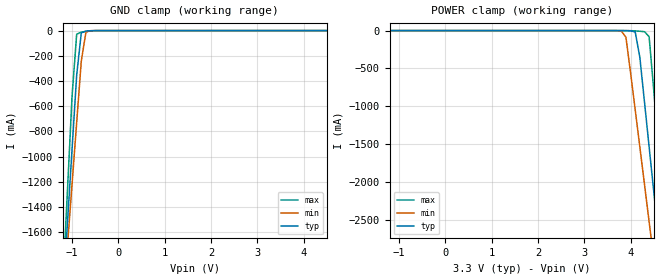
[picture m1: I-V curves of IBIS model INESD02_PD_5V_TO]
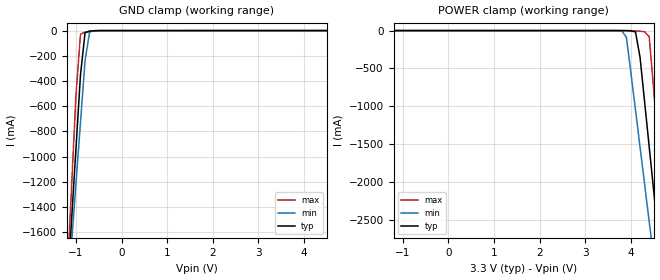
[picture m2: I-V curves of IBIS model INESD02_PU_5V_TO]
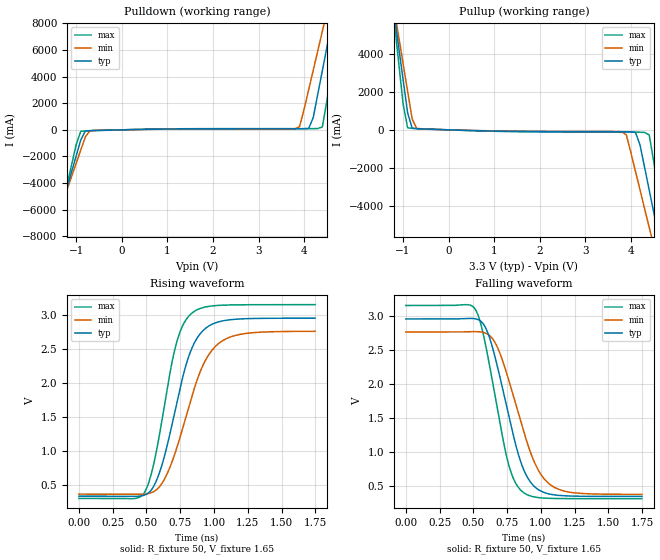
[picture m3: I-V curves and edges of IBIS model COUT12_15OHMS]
|   This file is an IBIS representation of the   |
|   Integrated Device Technology, Inc.   |
|   ICS810252i-02   |
[IBIS Ver]   4.1
[File name]   810252di_02_3v3.ibs
[File Rev]   1.0
[Date]   28 Apr 2009 | Last modified
|   Nov 27 2007  | Generated
[Source]   Originated at Integrated Devices Technology, Inc.
[Disclaimer]
IDT hereby grants the user of this IBIS model a non-exclusive,
nontransferable license to use this IBIS model under the following terms.
Before using this IBIS model, the user should read this license.
If the user does not accept these terms,  the IBIS model should be
returned to IDT within 30 days.
   The user is granted this license only to use the IBIS model and
is not granted rights to sell, load, rent, lease or license the IBIS
model in whole or in part, or in modified form to anyone other than
user. User may modify the IBIS model to suit its specific
applications but rights to derivative works and such modifications
shall belong to IDT.
   This IBIS model is provided on an "AS IS" basis and IDT makes
absolutely no warranty with respect to the information contained
herein. IDT DISCLAIMS AND CUSTOMER WAIVES ALL WARRANTIES, EXPRESS
OR IMPLIED, INCLUDING WARRANTIES OF MERCHANTABILITY OR FITNESS FOR
A PARTICULAR PURPOSE. The entire risk as to quality and performance
is with the Customer. ACCORDINGLY, IN NO EVENT SHALL THE COMPANY BE
LIABLE FOR ANY DAMAGES, WHETHER IN CONTRACT OR TORT,INCLUDING ANY
LOST PROFITS OR OTHER INCIDENTAL, CONSEQUENTIAL, EXEMPLARY, OR
PUNITIVE DAMAGES ARISING OUT OF THE USE OR APPLICATION OF THE IBIS
model provided in this package. Further, IDT reserves the right to
make changes without notice to any product herein to improve
reliability, function, or design. IDT does not convey any license
under patent rights or any other intellectual property rights,
including those of third parties.
   IDT is not obligated to provide maintenance or support
for the licensed IBIS model.
[Copyright]   Copyright 2007 by Integrated Device Technology, Inc.
[Component]   ICS810252DKI-02
[Manufacturer] Integrated Devices Technology, Inc.
[Package]
|QFN 32
|lead + wire   typ   min   max
R_pkg   72.4655m   58.886m   86.045m
L_pkg   1.47175nH   1.11650nH   1.77850nH
C_pkg   0.07747pF   0.07444pF   0.08050pF
[Pin] signal_name   model_name   R_pin   L_pin   C_pin
1   LF1   NC   86.045m   1.77850nH   0.08050pF
2   LF0   NC   76.996m   1.55783nH   0.07848pF
3   ISET   NC   67.941m   1.33717nH   0.07646pF
4   GND   GND   58.886m   1.11650nH   0.07444pF
5   CLK_SEL   INESD02_PD_5V_TO   58.886m   1.11650nH   0.07444pF
6   VDD   POWER   67.941m   1.33717nH   0.07646pF
7   RESERVED   NC   76.996m   1.55783nH   0.07848pF
8   GND   GND   86.045m   1.77850nH   0.08050pF
9   PDSEL_2   INESD02_PU_5V_TO   86.045m   1.77850nH   0.08050pF
10   PDSEL_1   INESD02_PU_5V_TO   76.996m   1.55783nH   0.07848pF
11   PDSEL_0   INESD02_PU_5V_TO   67.941m   1.33717nH   0.07646pF
12   VDD   POWER   58.886m   1.11650nH   0.07444pF
13   VDDA   POWER   58.886m   1.11650nH   0.07444pF
14   ODBSEL_1   INESD02_PD_5V_TO   67.941m   1.33717nH   0.07646pF
15   ODBSEL_0   INESD02_PD_5V_TO   76.996m   1.55783nH   0.07848pF
16   ODASEL_1   INESD02_PD_5V_TO   86.045m   1.77850nH   0.08050pF
17   ODASEL_0   INESD02_PD_5V_TO   86.045m   1.77850nH   0.08050pF
18   GND   GND   76.996m   1.55783nH   0.07848pF
19   QA   COUT12_15OHMS   67.941m   1.33717nH   0.07646pF
20   NC   NC   58.886m   1.11650nH   0.07444pF
21   VDDO   POWER   58.886m   1.11650nH   0.07444pF
22   QB   COUT12_15OHMS   67.941m   1.33717nH   0.07646pF
23   NC   NC   76.996m   1.55783nH   0.07848pF
24   GND   GND   86.045m   1.77850nH   0.08050pF
25   nCLK1   INESD02_PMID_5V_   86.045m   1.77850nH   0.08050pF
26   CLK1   INESD02_PD_5V_TO   76.996m   1.55783nH   0.07848pF
27   VDD   POWER   67.941m   1.33717nH   0.07646pF
28   nCLK0   INESD02_PMID_5V_   58.886m   1.11650nH   0.07444pF
29   CLK0   INESD02_PD_5V_TO   58.886m   1.11650nH   0.07444pF
30   XTAL_OUT   NC   67.941m   1.33717nH   0.07646pF
31   XTAL_IN   NC   76.996m   1.55783nH   0.07848pF
32   VDDX   POWER   86.045m   1.77850nH   0.08050pF
| Models and submodels in the file (4): INESD02_PD_5V_TO (Input), INESD02_PU_5V_TO (Input), COUT12_15OHMS (Output), INESD02_PMID_5V_ (Input)
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[Model]   INESD02_PD_5V_TO
Model_type   Input
Polarity   Non-Inverting
Vinl = 0.8V
Vinh = 2.0V
|   typ   min   max
C_comp   2pF   1.5pF   2.5pF
|   typ   min   max
[Voltage range]  3.3V   3.135V   3.465V
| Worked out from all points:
|   GND clamp passes 1 mA (typ) near -0.60 V on its own axis
[GND_clamp]
|Voltage I(typ)   I(min)   I(max)
-3.3V     -14.52A    -12.53A    -17.87A
-1.2V     -2.123A    -2.201A    -2.031A
-1.1V     -1.533A    -1.71A     -1.276A
-1V       -943mA     -1.22A     -522mA
-900mV    -353.5mA   -729.8mA   -28.69mA
-800mV    -17.79mA   -240.3mA   -12.18mA
-700mV    -3.491mA   -12mA      -6.618mA
-600mV    -1.033mA   -835uA     -2.43mA
6.6V      128.6uA    160.8uA    121.8uA
[POWER_clamp]
|Voltage   I(typ)   I(min)   I(max)
-3.3V     128.6uA    156.8uA    124.8uA
3.8V      -180.1uA   -4.403mA   -11.05uA
3.9V      -1.033mA   -88.76mA   -99.86uA
4.1V      -17.79mA   -1.048A    -3.685mA
4.2V      -353.5mA   -1.539A    -8.437mA
4.3V      -943mA     -2.029A    -14.61mA
4.4V      -1.533A    -2.52A     -80.08mA
4.5V      -2.123A    -3.011A    -786mA
4.6V      -2.713A    -3.502A    -1.54A
4.7V      -3.303A    -3.994A    -2.295A
4.8V      -3.894A    -4.485A    -3.049A
6.6V      -14.52A    -13.34A    -16.62A
[Model]   INESD02_PU_5V_TO
Model_type   Input
Polarity   Non-Inverting
Vinl = 1.4V
Vinh = 1.85V
|   typ   min   max
C_comp   2pF   1.5pF   2.5pF
|   typ   min   max
[Voltage range]  3.3V   3.135V   3.465V
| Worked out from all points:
|   GND clamp passes 1 mA (typ) near -0.59 V on its own axis
[GND_clamp]
|Voltage   I(typ)   I(min)   I(max)
-3.3V     -14.52A    -12.53A    -17.87A
-1.2V     -2.123A    -2.201A    -2.031A
-1.1V     -1.533A    -1.71A     -1.276A
-1V       -943mA     -1.22A     -522.1mA
-900mV    -353.6mA   -729.9mA   -28.76mA
-800mV    -17.85mA   -240.4mA   -12.24mA
-700mV    -3.555mA   -12.08mA   -6.682mA
-600mV    -1.097mA   -911.4uA   -2.494mA
6.6V      64.29uA    84.42uA    57.85uA
[POWER_clamp]
|Voltage   I(typ)   I(min)   I(max)
-3.3V     64.29uA    80.4uA     60.89uA
3.8V      -244.4uA   -4.479mA   -74.98uA
3.9V      -1.097mA   -88.84mA   -163.8uA
4.1V      -17.85mA   -1.048A    -3.749mA
4.2V      -353.6mA   -1.539A    -8.501mA
4.3V      -943mA     -2.029A    -14.67mA
4.4V      -1.533A    -2.52A     -80.15mA
4.5V      -2.123A    -3.011A    -786mA
4.6V      -2.713A    -3.502A    -1.54A
4.7V      -3.303A    -3.994A    -2.295A
4.8V      -3.894A    -4.485A    -3.049A
6.6V      -14.52A    -13.34A    -16.62A
[Model]   COUT12_15OHMS
Model_type   Output
Polarity   Non-Inverting
|   typ   min   max
C_comp   2pF   1.5pF   2.5pF
Vmeas = 1.65V
Rref = 50
Cref = 0
Vref = 1.65V
|   typ   min   max
[Voltage range]   3.3V   3.135V   3.465V
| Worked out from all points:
|   slope of the pulldown table from 0 to 0.495 V, typ, clamps not added: 13.8 ohm
|   slope of the pullup table from 0 to 0.495 V, typ, clamps not added: 13.7 ohm
|   rising waveform, R_fixture 50, V_fixture 1.65: 20-80 % time 196ps typ, 233ps min, 161ps max; typ from 0.341 V to 2.96 V
|   falling waveform, R_fixture 50, V_fixture 1.65: 20-80 % time 193ps typ, 225ps min, 163ps max; typ from 2.96 V to 0.341 V
[Pulldown]
|Voltage   I (typ)   I (min)   I (max)
-3.3V     -29.16A    -25.19A    -35.83A
-1.5V     -7.869A    -7.438A    -8.66A
-1.4V     -6.685A    -6.452A    -7.149A
-900mV    -768.5mA   -1.522A    -115.3mA
-700mV    -59.09mA   -73.31mA   -66.33mA
3.9V      79.76mA    237.3mA    91.46mA
4.2V      910.1mA    4.459A     92.62mA
4.4V      4.426A     7.39A      211.8mA
4.6V      7.945A     10.32A     4.422A
4.7V      9.706A     11.79A     6.671A
4.8V      11.47A     13.26A     8.921A
6.6V      43.31A     39.79A     49.6A
[Pullup]
|Voltage   I (typ)   I (min)   I (max)
-3.3V     43.25A     37.32A     53.22A
-1.2V     6.19A      6.441A     5.891A
-1.1V     4.426A     4.972A     3.638A
-900mV    900.3mA    2.035A     106.9mA
-700mV    58.42mA    71.68mA    66.98mA
3.8V      -101.6mA   -99.35mA   -118.6mA
4.1V      -137.6mA   -2.195A    -121.4mA
4.3V      -1.989A    -4.161A    -136.8mA
4.4V      -3.169A    -5.144A    -265.7mA
4.6V      -5.53A     -7.113A    -3.183A
4.8V      -7.892A    -9.082A    -6.199A
6.6V      -29.16A    -26.81A    -33.35A
[Ramp]
|   typ   min   max
dV/dt_r   2.093/0.305n   1.914/0.364n   2.279/0.249n
dV/dt_f   2.098/0.289n   1.918/0.339n   2.286/0.243n
R_load =   50.0000
[Rising Waveform]
R_fixture = 50
V_fixture = 1.65   |Vcc_typ
V_fixture_min = 1.5675 |Vcc_min
V_fixture_max = 1.7325 |Vcc_max
C_fixture = 0.0p
| Time   typ   min   max
0s        340.7mV    370.7mV    307.4mV
487ps     357.9mV    371.6mV    399.2mV
537.8ps   436.5mV    393.1mV    680.8mV
593.8ps   670.5mV    472.7mV    1.213V
718.2ps   1.65V      1.01V      2.56V
770.8ps   2.104V     1.354V     2.855V
837.3ps   2.518V     1.812V     3.031V
947.7ps   2.821V     2.374V     3.124V
1.083ns   2.922V     2.645V     3.147V
1.748ns   2.955V     2.762V     3.153V
[Falling Waveform]
R_fixture = 50
V_fixture = 1.65   |Vcc_typ
V_fixture_min = 1.5675 |Vcc_min
V_fixture_max = 1.7325 |Vcc_max
C_fixture = 0.0p
| Time   typ   min   max
0s        2.955V     2.763V     3.153V
515ps     2.957V     2.769V     3.095V
551.8ps   2.927V     2.764V     2.909V
593.8ps   2.814V     2.743V     2.543V
670.9ps   2.315V     2.569V     1.715V
767.3ps   1.49V      2.021V     771.3mV
865.4ps   772.6mV    1.349V     407mV
975.7ps   448.5mV    748.1mV    324.9mV
1.098ns   363.7mV    476.5mV    310.5mV
1.748ns   340.8mV    371.1mV    307.4mV
